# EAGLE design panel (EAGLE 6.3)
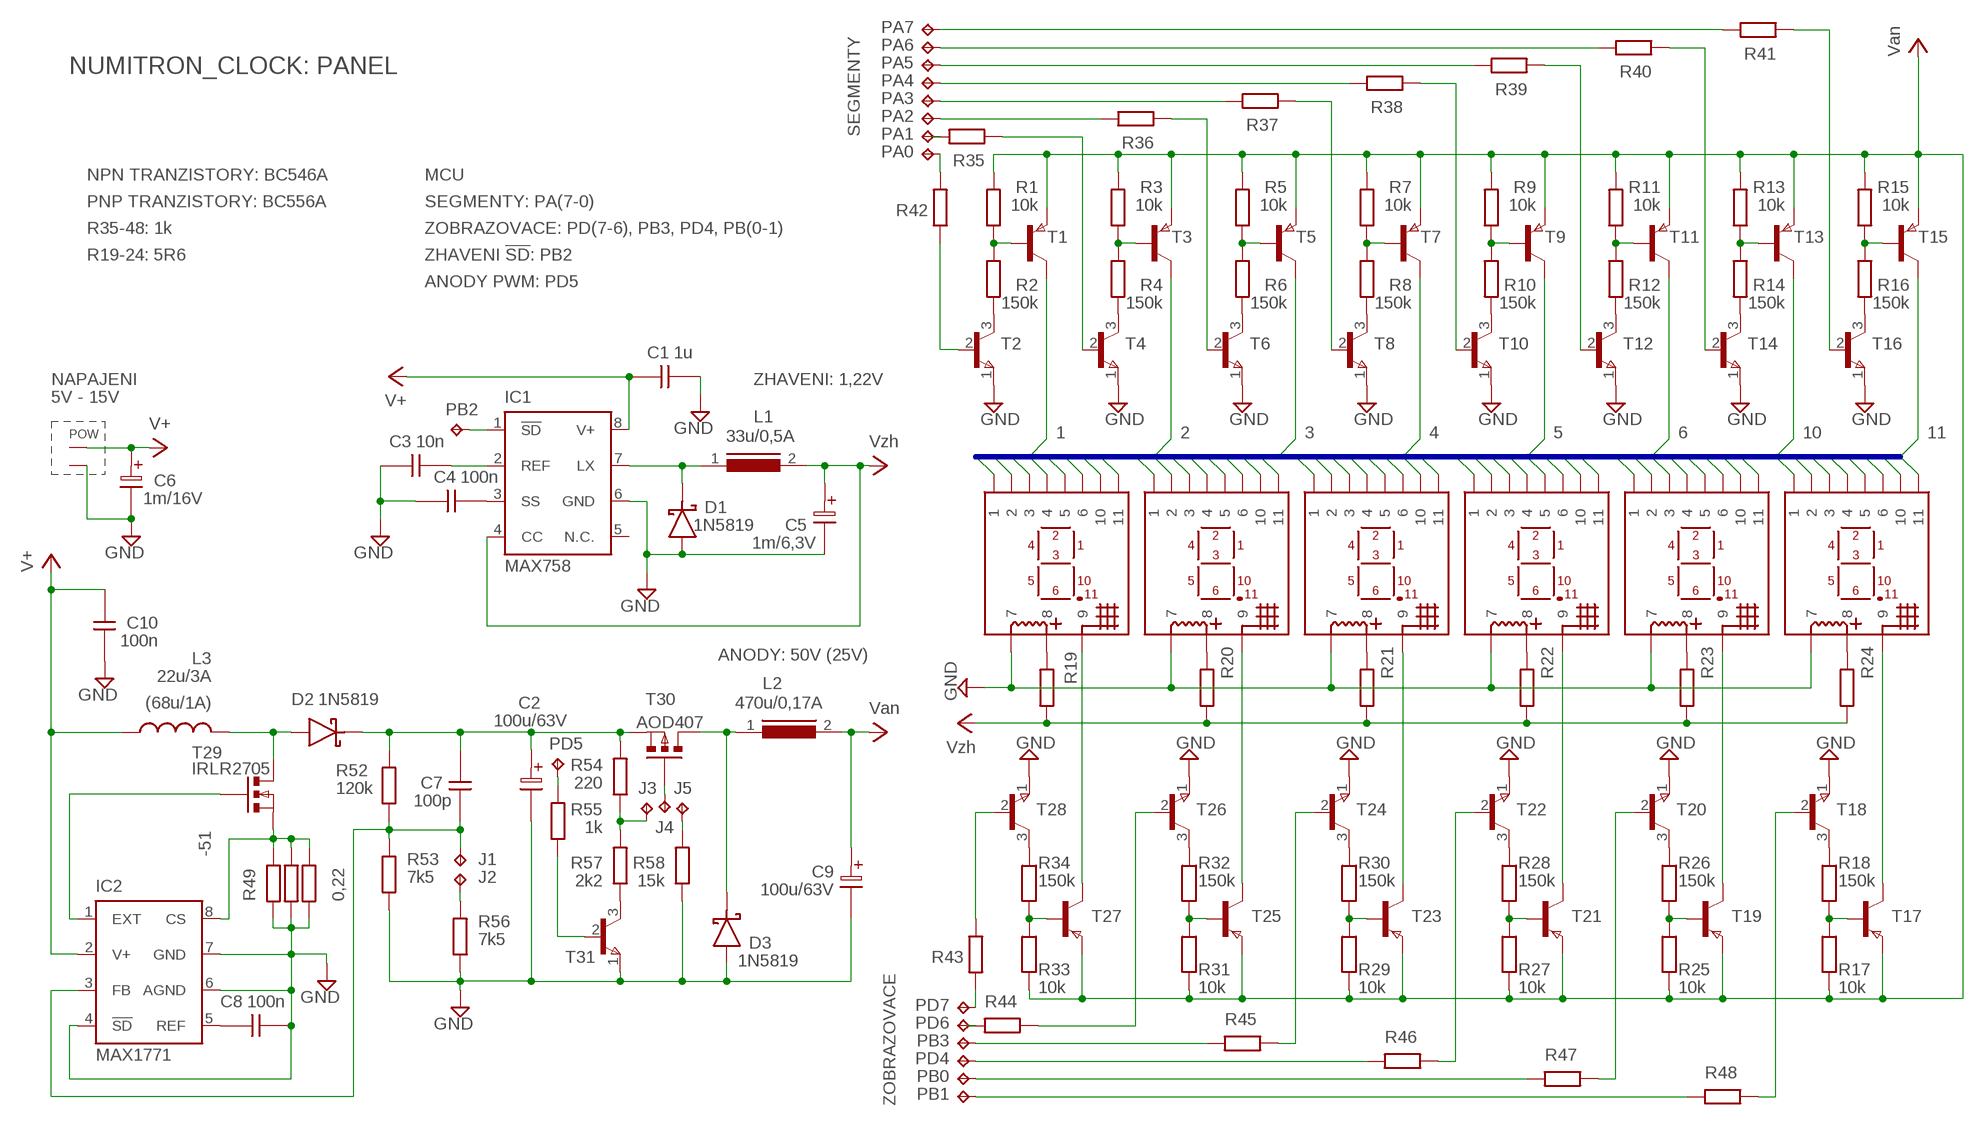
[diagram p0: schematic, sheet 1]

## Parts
C1  1u  CK  [CK]
C2  100u/63V  CT15  [CT15]
C3  10n  CK  [CK]
C4  100n  CK  [CK]
C5  1m/6,3V  CT15  [CT15]
C6  1m/16V  CT15  [CT15]
C7  100p  CK  [CK]
C8  100n  CK  [CK]
C9  100u/63V  CT15  [CT15]
C10  100n  CK  [CK]
D1  1N5819  [DO41]
D2  1N5819  [DO41]
D3  1N5819  [DO41]
DIGIT1  IV6  [IV6]
DIGIT2  IV6  [IV6]
DIGIT3  IV6  [IV6]
DIGIT4  IV6  [IV6]
DIGIT5  IV6  [IV6]
DIGIT6  IV6  [IV6]
IC1  MAX758  [DIL08]
IC2  MAX1771  [DIL08]
J1  TPPAD1-13Y  [P1-13Y]
J2  TPPAD1-13Y  [P1-13Y]
J3  TPPAD1-13Y  [P1-13Y]
J4  TPPAD1-13Y  [P1-13Y]
J5  TPPAD1-13Y  [P1-13Y]
L1  33u/0,5A  SMCC12  [SMCC12]
L2  470u/0,17A  SMCC12  [SMCC12]
L3  22u/3A  TOR.  [L_14X8]
PA0  TPPAD1-13Y  [P1-13Y]
PA1  TPPAD1-13Y  [P1-13Y]
PA2  TPPAD1-13Y  [P1-13Y]
PA3  TPPAD1-13Y  [P1-13Y]
PA4  TPPAD1-13Y  [P1-13Y]
PA5  TPPAD1-13Y  [P1-13Y]
PA6  TPPAD1-13Y  [P1-13Y]
PA7  TPPAD1-13Y  [P1-13Y]
PB0  TPPAD1-13Y  [P1-13Y]
PB1  TPPAD1-13Y  [P1-13Y]
PB2  TPPAD1-13Y  [P1-13Y]
PB3  TPPAD1-13Y  [P1-13Y]
PD4  TPPAD1-13Y  [P1-13Y]
PD5  TPPAD1-13Y  [P1-13Y]
PD6  TPPAD1-13Y  [P1-13Y]
PD7  TPPAD1-13Y  [P1-13Y]
POW  ARK500/2  [ARK500/2]
R1  10k  MRRB  [MRR_1206]
R2  150k  MRRB  [MRR_1206]
R3  10k  MRRB  [MRR_1206]
R4  150k  MRRB  [MRR_1206]
R5  10k  MRRB  [MRR_1206]
R6  150k  MRRB  [MRR_1206]
R7  10k  MRRB  [MRR_1206]
R8  150k  MRRB  [MRR_1206]
R9  10k  MRRB  [MRR_1206]
R10  150k  MRRB  [MRR_1206]
R11  10k  MRRB  [MRR_1206]
R12  150k  MRRB  [MRR_1206]
R13  10k  MRRB  [MRR_1206]
R14  150k  MRRB  [MRR_1206]
R15  10k  MRRB  [MRR_1206]
R16  150k  MRRB  [MRR_1206]
R17  10k  MRRB  [MRR_1206]
R18  150k  MRRB  [MRR_1206]
R19  MRRB  [MRR_1206]
R20  MRR'  [MRR]
R21  MRR'  [MRR]
R22  MRRA  [MRR_0204/10]
R23  MRRA  [MRR_0204/10]
R24  MRRA  [MRR_0204/10]
R25  10k  MRRB  [MRR_1206]
R26  150k  MRRB  [MRR_1206]
R27  10k  MRRB  [MRR_1206]
R28  150k  MRRB  [MRR_1206]
R29  10k  MRRB  [MRR_1206]
R30  150k  MRRB  [MRR_1206]
R31  10k  MRRB  [MRR_1206]
R32  150k  MRRB  [MRR_1206]
R33  10k  MRRB  [MRR_1206]
R34  150k  MRRB  [MRR_1206]
R35  MRR'  [MRR]
R36  MRR'  [MRR]
R37  MRR'  [MRR]
R38  MRR'  [MRR]
R39  MRR'  [MRR]
R40  MRR'  [MRR]
R41  MRR'  [MRR]
R42  MRR'  [MRR]
R43  MRR'  [MRR]
R44  MRR'  [MRR]
R45  MRR'  [MRR]
R46  MRR'  [MRR]
R47  MRR'  [MRR]
R48  MRR'  [MRR]
R49  0,22  MRR-10  [RR-10]
R50  0,22  MRR-10  [RR-10]
R51  0,22  MRR-10  [RR-10]
R52  120k  MRR'  [MRR]
R53  7k5  MRR'  [MRR]
R54  220  MRR'  [MRR]
R55  1k  MRR'  [MRR]
R56  7k5  MRR'  [MRR]
R57  2k2  MRR'  [MRR]
R58  15k  MRR'  [MRR]
T1  BC556  BC556A  [TO-92C]
T2  BC546  BC546A  [TO-92C]
T3  BC546  BC556A  [TO-92C]
T4  BC546  BC546A  [TO-92C]
T5  BC546  BC556A  [TO-92C]
T6  BC546  BC546A  [TO-92C]
T7  BC546  BC556A  [TO-92C]
T8  BC546  BC546A  [TO-92C]
T9  BC546  BC556A  [TO-92C]
T10  BC546  BC546A  [TO-92C]
T11  BC546  BC556A  [TO-92C]
T12  BC546  BC546A  [TO-92C]
T13  BC546  BC556A  [TO-92C]
T14  BC546  BC546A  [TO-92C]
T15  BC546  BC556A  [TO-92C]
T16  BC546  BC546A  [TO-92C]
T17  BC546  BC556A  [TO-92C]
T18  BC546  BC546A  [TO-92C]
T19  BC546  BC556A  [TO-92C]
T20  BC546  BC546A  [TO-92C]
T21  BC546  BC556A  [TO-92C]
T22  BC546  BC546A  [TO-92C]
T23  BC546  BC556A  [TO-92C]
T24  BC546  BC546A  [TO-92C]
T25  BC546  BC556A  [TO-92C]
T26  BC546  BC546A  [TO-92C]
T27  BC546  BC556A  [TO-92C]
T28  BC546  BC546A  [TO-92C]
T29  IRLR2705  IRF540  [D2PAK]
T30  AOD407  IRF9540  [D2PAK]
T31  BC546  BC546A  [TO-92C]

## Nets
GND: C1.2 C2.2 C3.1 C4.1 C5.2 C6.2 C8.2 C9.2 C10.1 D1.A D3.A DIGIT1.P$7 DIGIT2.P$7 DIGIT3.P$7 DIGIT4.P$7 DIGIT5.P$7 DIGIT6.P$7 IC1.6(GND) IC2.4(!SD) IC2.6(AGND) IC2.7(GND) POW.2 R49.1 R50.1 R51.1 R53.2 R56.2 R58.1 T2.1(E) T4.1(E) T6.1(E) T8.1(E) T10.1(E) T12.1(E) T14.1(E) T16.1(E) T18.1(E) T20.1(E) T22.1(E) T24.1(E) T26.1(E) T28.1(E) T31.1(E)
N$1: R1.1 R2.2 T1.2(B)
N$2: R2.1 T2.3(C)
N$3: J2.TP R56.1
N$4: R3.1 R4.2 T3.2(B)
N$5: R4.1 T4.3(C)
N$6: PA0.TP R42.1
N$7: R5.1 R6.2 T5.2(B)
N$8: R6.1 T6.3(C)
N$9: PA1.TP R35.2
N$10: R7.1 R8.2 T7.2(B)
N$11: R8.1 T8.3(C)
N$12: PA2.TP R36.2
N$13: R9.1 R10.2 T9.2(B)
N$14: R10.1 T10.3(C)
N$15: PA3.TP R37.2
N$16: R11.1 R12.2 T11.2(B)
N$17: R12.1 T12.3(C)
N$18: PA4.TP R38.2
N$19: R13.1 R14.2 T13.2(B)
N$20: R14.1 T14.3(C)
N$21: PA5.TP R39.2
N$22: R15.1 R16.2 T15.2(B)
N$23: R16.1 T16.3(C)
N$24: PA6.TP R40.2
N$25: R17.1 R18.2 T17.2(B)
N$26: R18.1 T18.3(C)
N$27: PA7.TP R41.2
N$28: IC2.8(CS) R49.2 R50.2 R51.2 T29.S
N$29: DIGIT1.P$8 R19.2
N$30: DIGIT2.P$8 R20.2
N$31: DIGIT3.P$8 R21.2
N$32: DIGIT4.P$8 R22.2
N$33: DIGIT5.P$8 R23.2
N$34: DIGIT6.P$8 R24.2
N$35: IC1.1(!SD) PB2.TP
N$36: R25.1 R26.2 T19.2(B)
N$37: R26.1 T20.3(C)
N$38: R35.1 T4.2(B)
N$39: R27.1 R28.2 T21.2(B)
N$40: R28.1 T22.3(C)
N$41: R36.1 T6.2(B)
N$42: R29.1 R30.2 T23.2(B)
N$43: R30.1 T24.3(C)
N$44: R37.1 T8.2(B)
N$45: R31.1 R32.2 T25.2(B)
N$46: R32.1 T26.3(C)
N$47: R38.1 T10.2(B)
N$48: R33.1 R34.2 T27.2(B)
N$49: R34.1 T28.3(C)
N$50: R39.1 T12.2(B)
N$51: DIGIT6.P$9 T17.3(C)
N$52: DIGIT5.P$9 T19.3(C)
N$53: DIGIT4.P$9 T21.3(C)
N$54: DIGIT3.P$9 T23.3(C)
N$55: DIGIT2.P$9 T25.3(C)
N$56: DIGIT1.P$9 T27.3(C)
N$57: R40.1 T14.2(B)
N$58: R42.2 T2.2(B)
N$59: R41.1 T16.2(B)
N$60: PD7.TP R43.2
N$61: R43.1 T28.2(B)
N$62: PD6.TP R44.1
N$63: PB3.TP R45.1
N$64: PD4.TP R46.1
N$65: PB0.TP R47.1
N$66: PB1.TP R48.1
N$67: R48.2 T18.2(B)
N$68: R47.2 T20.2(B)
N$69: R46.2 T22.2(B)
N$70: R45.2 T24.2(B)
N$71: R44.2 T26.2(B)
N$72: J5.TP R58.2
N$73: C4.2 IC1.3(SS)
N$74: D1.K IC1.7(LX) L1.1
N$75: C3.2 IC1.2(REF)
N$76: IC2.1(EXT) T29.G
N$77: R55.1 T31.2(B)
N$78: D2.A L3.P$4 T29.D
N$79: C7.1 IC2.3(FB) J1.TP R52.2 R53.1
N$80: C2.1 C7.2 D2.K R52.1 R54.2 T30.S
N$81: D3.K L2.1 T30.D
N$82: J4.TP T30.G
N$83: R57.1 T31.3(C)
N$84: PD5.TP R55.2
N$85: J3.TP R54.1 R57.2
N$87: C8.1 IC2.5(REF)
SEGMENTY0: DIGIT1.P$1 DIGIT2.P$1 DIGIT3.P$1 DIGIT4.P$1 DIGIT5.P$1 DIGIT6.P$1 T1.3(C)
SEGMENTY1: DIGIT1.P$2 DIGIT2.P$2 DIGIT3.P$2 DIGIT4.P$2 DIGIT5.P$2 DIGIT6.P$2 T3.3(C)
SEGMENTY2: DIGIT1.P$3 DIGIT2.P$3 DIGIT3.P$3 DIGIT4.P$3 DIGIT5.P$3 DIGIT6.P$3 T5.3(C)
SEGMENTY3: DIGIT1.P$4 DIGIT2.P$4 DIGIT3.P$4 DIGIT4.P$4 DIGIT5.P$4 DIGIT6.P$4 T7.3(C)
SEGMENTY4: DIGIT1.P$5 DIGIT2.P$5 DIGIT3.P$5 DIGIT4.P$5 DIGIT5.P$5 DIGIT6.P$5 T9.3(C)
SEGMENTY5: DIGIT1.P$6 DIGIT2.P$6 DIGIT3.P$6 DIGIT4.P$6 DIGIT5.P$6 DIGIT6.P$6 T11.3(C)
SEGMENTY6: DIGIT1.P$10 DIGIT2.P$10 DIGIT3.P$10 DIGIT4.P$10 DIGIT5.P$10 DIGIT6.P$10 T13.3(C)
SEGMENTY7: DIGIT1.P$11 DIGIT2.P$11 DIGIT3.P$11 DIGIT4.P$11 DIGIT5.P$11 DIGIT6.P$11 T15.3(C)
V+: C1.1 C6.1 C10.2 IC1.8(V+) IC2.2(V+) L3.P$3 POW.1
VAN: C9.1 L2.2 R1.2 R3.2 R5.2 R7.2 R9.2 R11.2 R13.2 R15.2 R17.2 R25.2 R27.2 R29.2 R31.2 R33.2 T1.1(E) T3.1(E) T5.1(E) T7.1(E) T9.1(E) T11.1(E) T13.1(E) T15.1(E) T17.1(E) T19.1(E) T21.1(E) T23.1(E) T25.1(E) T27.1(E) ; supply symbol labelled Van
VZH: C5.1 IC1.4(CC) L1.2 R19.1 R20.1 R21.1 R22.1 R23.1 R24.1 ; supply symbol labelled Vzh
Unconnected: IC1.5(N.C.)

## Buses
SEGMENTY[0..7]

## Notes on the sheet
- NUMITRON_CLOCK: PANEL
- SEGMENTY
- NPN TRANZISTORY: BC546A | MCU
- PNP TRANZISTORY: BC556A | SEGMENTY: PA(7-0)
- R35-48: 1k | ZOBRAZOVACE: PD(7-6), PB3, PD4, PB(0-1)
- R19-24: 5R6 | ZHAVENI !SD!: PB2
- ANODY PWM: PD5
- NAPAJENI | ZHAVENI: 1,22V
- 5V - 15V
- 1 | 2 | 3 | 4 | 5 | 6 | 10 | 11
- ANODY: 50V (25V)
- (68u/1A)
- -51
- ZOBRAZOVACE

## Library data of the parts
C1 C3 C4 C7 C8 C10 = #_GM99:CK
C2 C5 C6 C9 = #_GM99:CT15: RM = 5mm, R = 10mm
D1-D3 = #_GM99:1N5819
DIGIT1-DIGIT6 = #_my:IV6
IC1 = #_my:MAX758
IC2 = #_my:MAX1771
J1-J5 PA0 PA1-PA7 PB0 PB1-PB3 PD4-PD7 = testpad:TP: Test pad
L1 L2 = inductors:SMCC12: INDUCTOR
L3 = #_my:TOR.
POW = #_GM99:ARK500/2
R1-R48 R52-R58 = #_GM99:MRR
R49-R51 = #_GM99:MRR-10
T1 T3 T5 T7 T9 T11 T13 T15 T17 T19 T21 T23 T25 T27 = #_GM99:BC556A
T2 T4 T6 T8 T10 T12 T14 T16 T18 T20 T22 T24 T26 T28 T31 = #_GM99:BC546A
T29 = #_my:IRF540
T30 = #_my:IRF9540

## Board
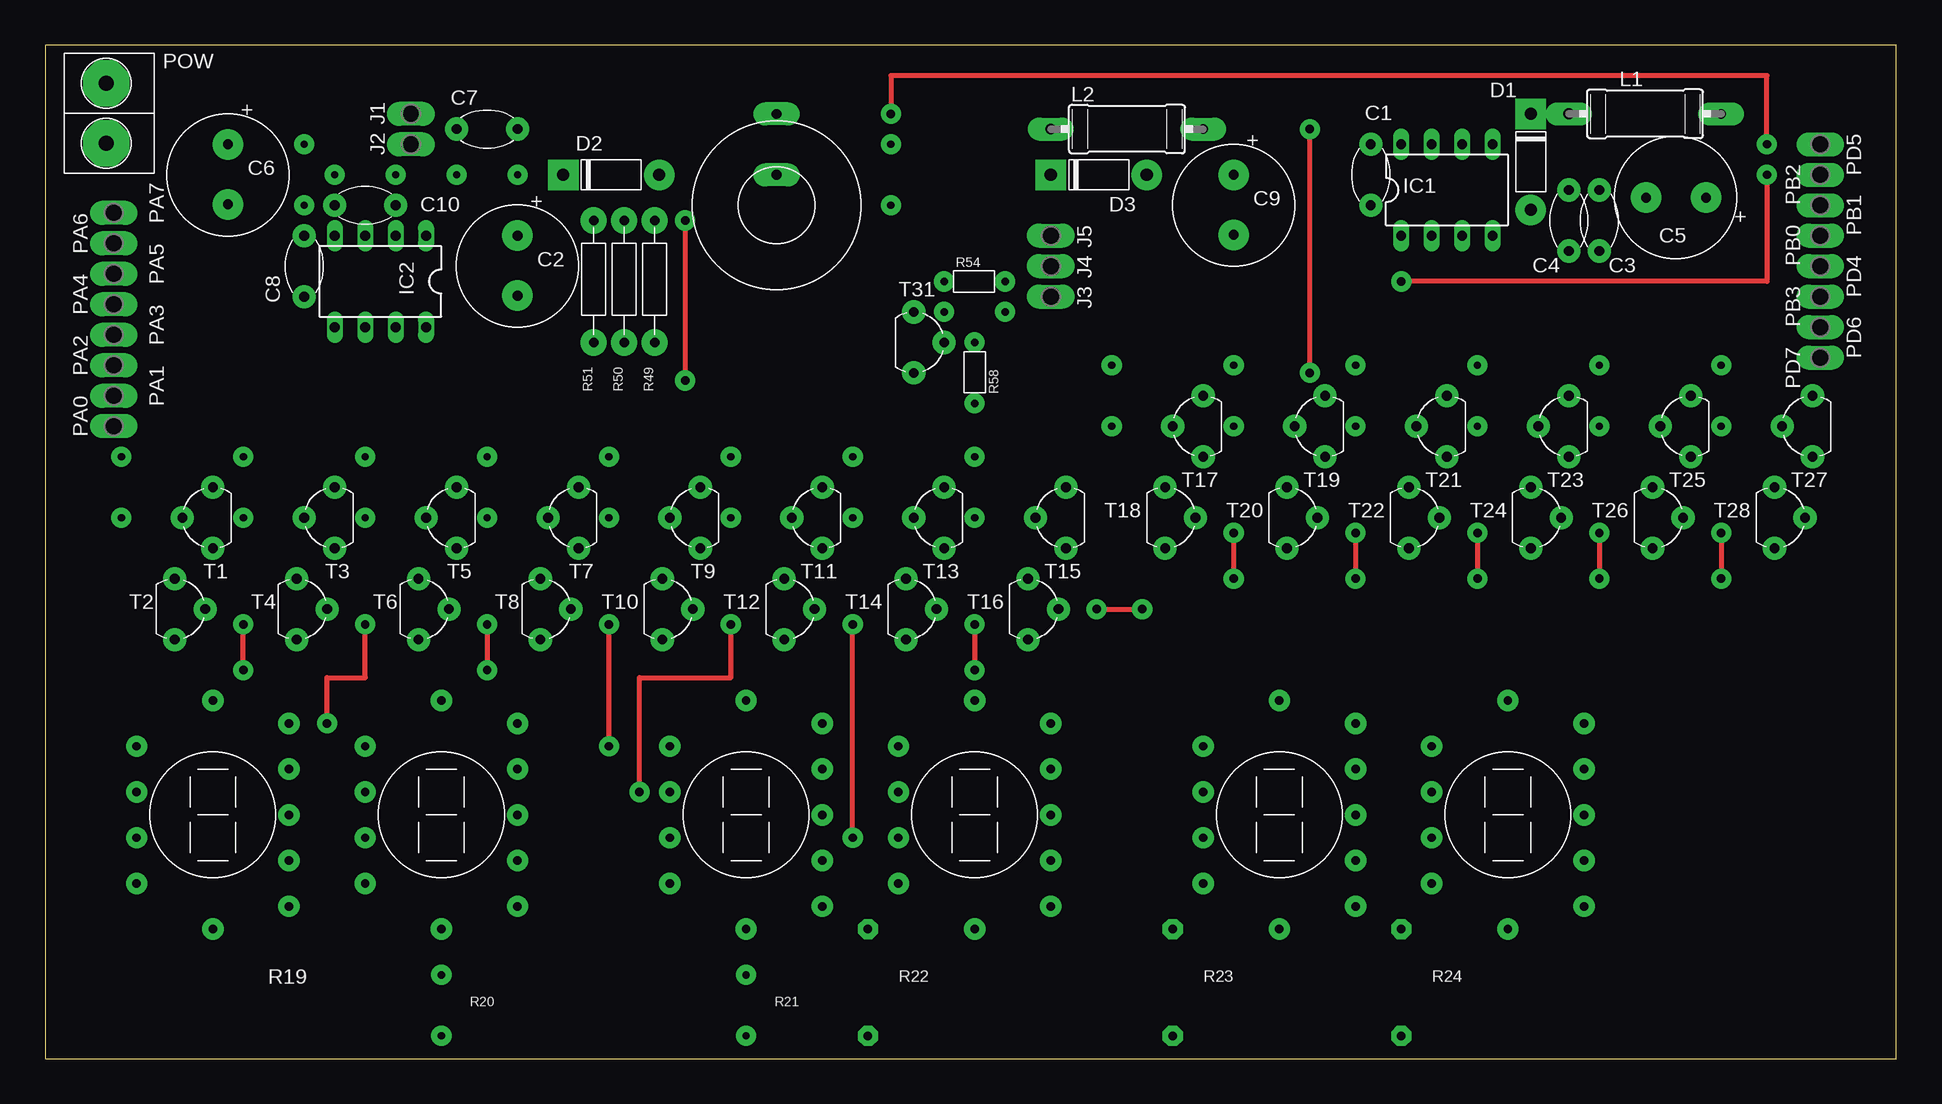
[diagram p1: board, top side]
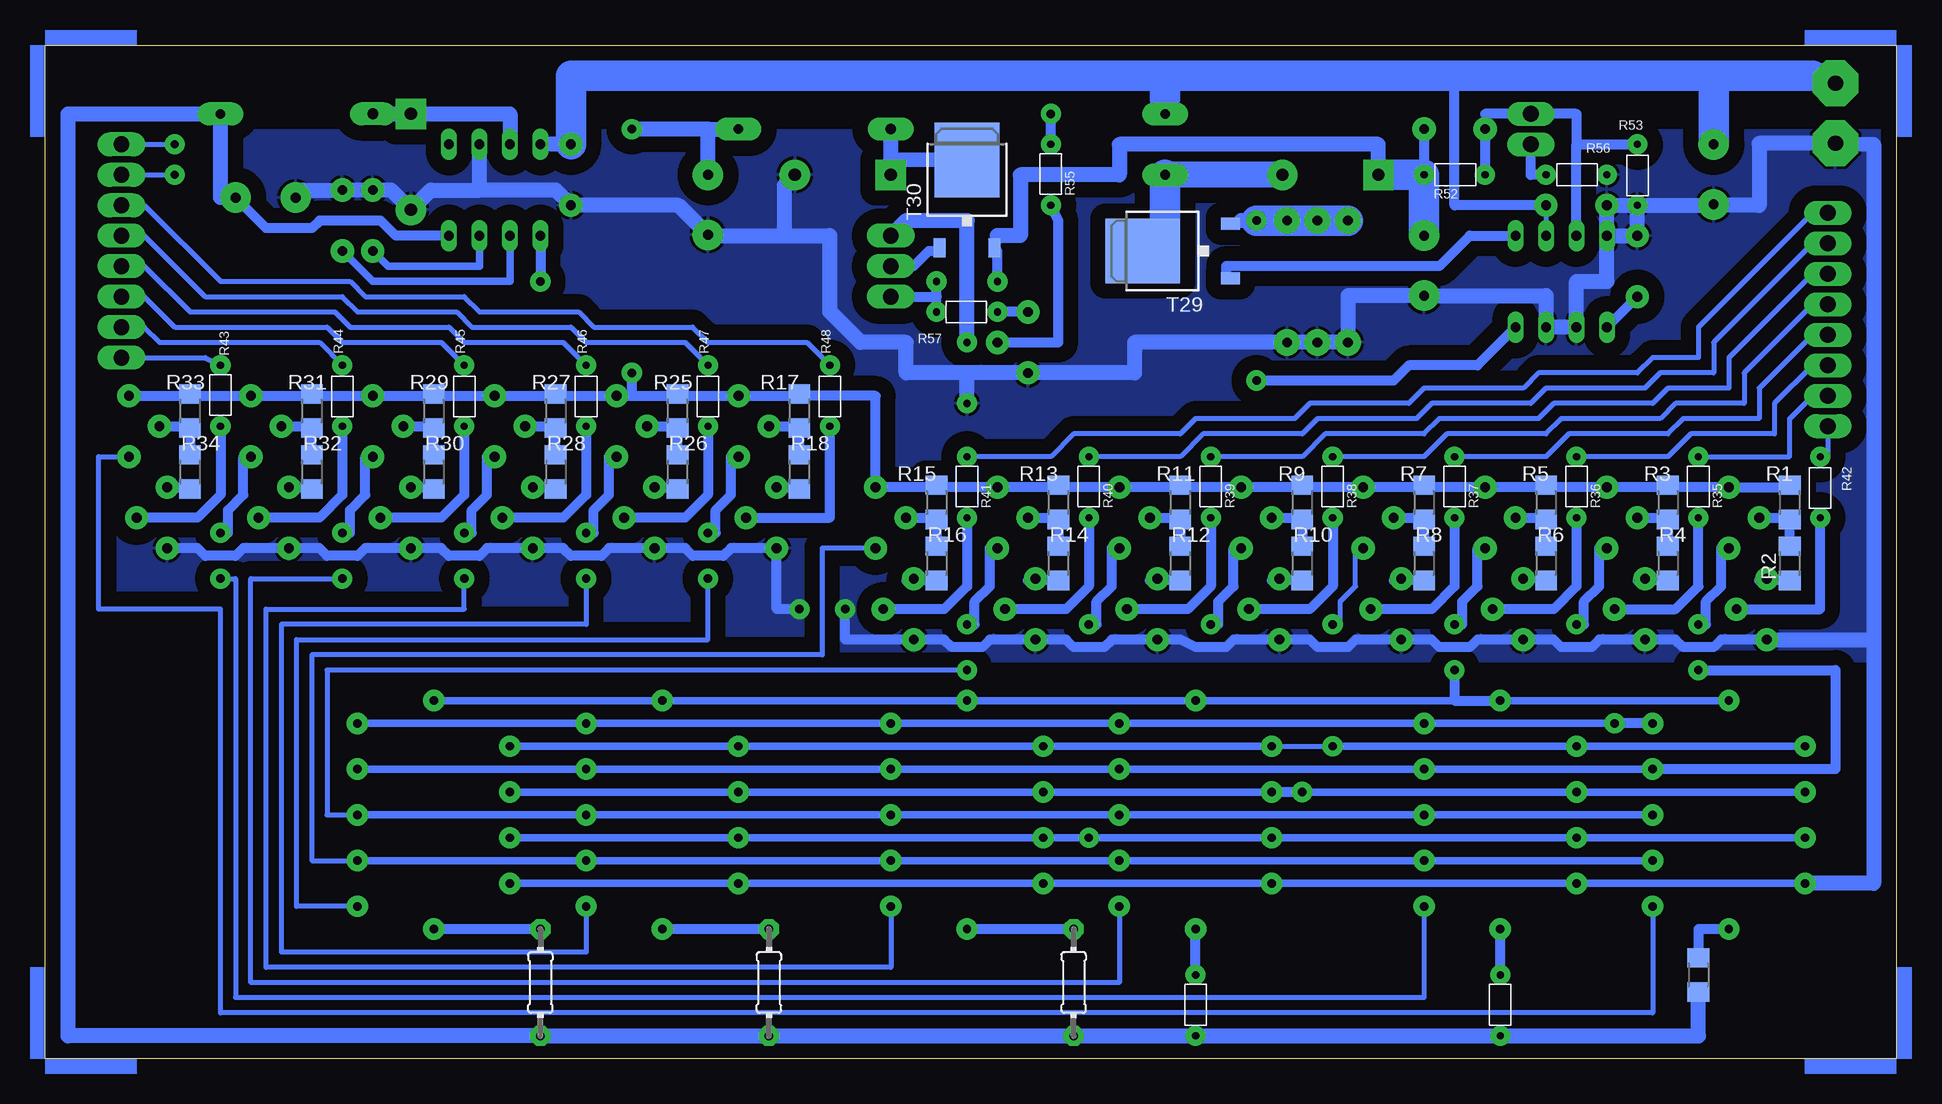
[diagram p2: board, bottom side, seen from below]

Size 154.31 x 84.45 mm. Coordinates in mm from the lower left corner, seen from the top.
Outline: 0,0 154.31,0 154.31,84.45 0,84.45 0,0
Copper layers (1*16): Top 0.035mm / dielectric 1.5mm / Bottom 0.035mm
Design rules "default": minimum track width 10mil, minimum drill 24mil, track to track 8mil, track to pad 8mil, pad to pad 8mil, via to via 8mil, smd to smd 8mil, copper to edge 40mil, drill to drill 8mil, minimum pad ring 10mil, minimum via ring 8mil, stop-mask expansion 4mil, vias tented up to drill 0mil, thermal gap 10mil

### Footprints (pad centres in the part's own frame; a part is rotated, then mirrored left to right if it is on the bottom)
CK = drill 0.813 pad 1.93: 1 0,0; 2 5.08,0
CT15 = drill 0.813 pad 2.54: 1 0,0; 2 5,0
DO41 = drill 1.016 pad 2.54: A 8,0 | drill 1.016 pad 2.54 square: K 0,0
IV6 = drill 0.7 pad 1.778: P$1 6.35,3.81; P$2 6.35,7.62; P$3 0,9.525; P$4 -6.35,5.715; P$5 -6.35,1.905; P$6 -6.35,-1.905; P$7 -6.35,-5.715; P$8 0,-9.525; P$9 6.35,-7.62; P$10 6.35,0; P$11 6.35,-3.81
DIL08 = drill 0.813 long: 1 -3.81,-3.81; 2 -1.27,-3.81; 3 1.27,-3.81; 4 3.81,-3.81; 5 3.81,3.81; 6 1.27,3.81; 7 -1.27,3.81; 8 -3.81,3.81
P1-13Y = drill 1.321 pad 1.905 long: TP 0,0
SMCC12 = drill 0.9 pad 1.93 long: 1 -6.35,0 | drill 0.8 pad 1.93 long: 2 6.35,0
L_14X8 = drill 0.8 pad 1.93 long: P$3 0,7.62; P$4 0,2.54
ARK500/2 = drill 1.27 pad 3.81 octagon: 1 0,0; 2 5,0
MRR_1206 = smd 1.6 x 1.803: 1 -1.422,0; 2 1.422,0
MRR = drill 0.61 pad 1.676: 1 0,0; 2 5.08,0
MRR_0204/10 = drill 0.7 pad 1.676 octagon: 1 -4.445,0; 2 4.445,0
RR-10 = drill 0.8 pad 2.184: 1 0,0; 2 10.16,0
TO-92C = drill 0.813 pad 1.93: 1 0,-1.27; 2 2.54,1.27; 3 0,3.81
D2PAK = smd 5.4 x 6.2: D 0,1.23 | smd 1 x 1.6: G -2.28,-6.07; S 2.28,-6.07

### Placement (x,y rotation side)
C1  110.49,76.2 270 top
C2  39.37,68.58 270 top
C3  129.54,72.39 270 top
C4  127,72.39 270 top
C5  138.43,71.75 180 top
C6  15.24,76.2 270 top
C7  34.29,77.47 0 top
C8  21.59,63.5 90 top
C9  99.06,73.66 270 top
C10  24.13,71.12 0 top
D1  123.83,78.74 270 top
D2  43.18,73.66 0 top
D3  83.82,73.66 0 top
DIGIT1  13.97,20.32 0 top
DIGIT2  33.02,20.32 0 top
DIGIT3  58.42,20.32 0 top
DIGIT4  77.47,20.32 0 top
DIGIT5  102.87,20.32 0 top
DIGIT6  121.92,20.32 0 top
IC1  116.84,72.39 0 top
IC2  27.94,64.77 180 top
J1  30.48,78.74 90 top
J2  30.48,76.2 90 top
J3  83.82,63.5 270 top
J4  83.82,66.04 270 top
J5  83.82,68.58 270 top
L1  133.35,78.74 0 top
L2  90.17,77.47 0 top
L3  60.96,71.12 0 top
PA0  5.71,52.7 90 top
PA1  5.71,55.24 90 top
PA2  5.71,57.78 90 top
PA3  5.71,60.33 90 top
PA4  5.71,62.87 90 top
PA5  5.71,65.41 90 top
PA6  5.71,67.94 90 top
PA7  5.71,70.48 90 top
PB0  147.96,68.58 270 top
PB1  147.96,71.12 270 top
PB2  147.96,73.66 270 top
PB3  147.96,63.5 270 top
PD4  147.96,66.04 270 top
PD5  147.96,76.2 270 top
PD6  147.96,60.96 270 top
PD7  147.96,58.42 270 top
POW  5.08,81.28 270 top
R1  8.89,46.35 90 bottom
R2  8.89,41.27 90 bottom
R3  19.05,46.35 90 bottom
R4  19.05,41.27 90 bottom
R5  29.21,46.35 90 bottom
R6  29.21,41.27 90 bottom
R7  39.37,46.35 90 bottom
R8  39.37,41.27 90 bottom
R9  49.53,46.35 90 bottom
R10  49.53,41.27 90 bottom
R11  59.69,46.35 90 bottom
R12  59.69,41.27 90 bottom
R13  69.85,46.35 90 bottom
R14  69.85,41.27 90 bottom
R15  80.01,46.35 90 bottom
R16  80.01,41.27 90 bottom
R17  91.44,53.98 90 bottom
R18  91.44,48.9 90 bottom
R19  16.51,6.99 90 bottom
R20  33.02,1.91 90 bottom
R21  58.42,1.91 90 bottom
R22  68.58,6.35 90 bottom
R23  93.98,6.35 90 bottom
R24  113.03,6.35 90 bottom
R25  101.6,53.98 90 bottom
R26  101.6,48.9 90 bottom
R27  111.76,53.98 90 bottom
R28  111.76,48.9 90 bottom
R29  121.92,53.98 90 bottom
R30  121.92,48.9 90 bottom
R31  132.08,53.98 90 bottom
R32  132.08,48.9 90 bottom
R33  142.24,53.98 90 bottom
R34  142.24,48.9 90 bottom
R35  16.51,45.09 90 bottom
R36  26.67,45.09 90 bottom
R37  36.83,45.09 90 bottom
R38  46.99,45.09 90 bottom
R39  57.15,45.09 90 bottom
R40  67.31,45.09 90 bottom
R41  77.47,45.09 90 bottom
R42  6.35,50.16 270 bottom
R43  139.7,52.7 90 bottom
R44  129.54,57.78 270 bottom
R45  119.38,57.78 270 bottom
R46  109.22,57.78 270 bottom
R47  99.06,57.78 270 bottom
R48  88.9,57.78 270 bottom
R49  50.8,59.69 90 top
R50  48.26,59.69 90 top
R51  45.72,59.69 90 top
R52  39.37,73.66 0 bottom
R53  21.59,76.2 270 bottom
R54  80.01,64.77 180 top
R55  70.48,71.12 90 bottom
R56  29.21,73.66 0 bottom
R57  74.93,62.23 180 bottom
R58  77.47,54.61 90 top
T1  13.97,46.35 180 top
T2  10.79,36.2 0 top
T3  24.13,46.35 180 top
T4  20.95,36.2 0 top
T5  34.29,46.35 180 top
T6  31.11,36.2 0 top
T7  44.45,46.35 180 top
T8  41.27,36.2 0 top
T9  54.61,46.35 180 top
T10  51.44,36.2 0 top
T11  64.77,46.35 180 top
T12  61.59,36.2 0 top
T13  74.93,46.35 180 top
T14  71.75,36.2 0 top
T15  85.09,46.35 180 top
T16  81.92,36.2 0 top
T17  96.52,53.98 180 top
T18  93.34,43.81 0 top
T19  106.68,53.98 180 top
T20  103.5,43.81 0 top
T21  116.84,53.98 180 top
T22  113.67,43.81 0 top
T23  127,53.98 180 top
T24  123.83,43.81 0 top
T25  137.16,53.98 180 top
T26  133.99,43.81 0 top
T27  147.32,53.98 180 top
T28  144.15,43.81 0 top
T29  61.59,67.31 90 bottom
T30  77.47,73.66 0 bottom
T31  72.39,58.42 0 top
U$1  [ANGLE-ARROW-NW1]  0,0 90 top
U$2  [ANGLE-ARROW-NW1]  0,84.45 0 top
U$3  [ANGLE-ARROW-NW1]  154.31,84.45 270 top
U$4  [ANGLE-ARROW-NW1]  154.31,0 180 top

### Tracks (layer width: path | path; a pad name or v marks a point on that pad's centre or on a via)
GND  (via drill 0.7 pad 1.68)
  Top 0.406: v87.63,37.47 v91.44,37.47
  Bottom 0.61: DIGIT1.P$7 DIGIT2.P$7 DIGIT3.P$7 DIGIT4.P$7 DIGIT5.P$7 DIGIT6.P$7
  Bottom 0.813: T28.1 141.6,42.55 140.97,41.91 138.43,41.91 137.79,42.55 T26.1 131.44,42.55 130.81,41.91 128.27,41.91 127.64,42.55 T24.1 121.28,42.55 120.65,41.91 118.11,41.91 117.47,42.55 T22.1 111.12,42.55 110.49,41.91 107.95,41.91 107.31,42.55 T20.1 100.97,42.55 100.33,41.91 97.79,41.91 97.16,42.55 T18.1 93.34,37.47 v91.44,37.47 | T2.1 14.61,34.92 15.24,34.29 17.78,34.29 18.41,34.92 T4.1 24.77,34.92 25.4,34.29 27.94,34.29 28.57,34.92 T6.1 34.92,34.92 35.56,34.29 38.1,34.29 38.73,34.92 T8.1 45.09,34.92 45.72,34.29 48.26,34.29 48.9,34.92 T10.1 55.24,34.92 55.88,34.29 58.42,34.29 59.69,34.92 T12.1 65.41,34.92 66.04,34.29 68.58,34.29 69.22,34.92 T14.1 75.56,34.92 76.2,34.29 78.74,34.29 79.38,34.92 T16.1 87.63,34.92 v87.63,37.47
  Bottom 1.27: T2.1 1.91,34.92 | 1.91,34.92 1.91,14.61 DIGIT1.P$7 | 1.91,34.92 1.91,76.2 POW.2 11.43,76.28 11.43,71.12 15.24,71.12 | R53.2 15.24,71.12 | 15.24,71.12 C6.2 | R53.2 C10.1 IC2.4 | R53.2 C8.2 IC2.4 | IC2.4 24.13,64.77 26.67,64.77 IC2.6 IC2.7 29.21,63.58 C2.2 45.72,63.58 R51.1 R50.1 R49.1 63.5,59.69 63.5,57.15 T31.1 77.47,57.15 | 77.47,57.15 82.55,57.15 82.55,59.69 86.36,59.69 88.9,62.23 88.9,68.58 92.71,68.58 | D3.A 92.71,72.77 92.71,68.58 | 92.71,68.58 98.98,68.58 C9.2 101.52,71.12 C1.2 111.76,72.39 118.11,72.39 | 118.11,72.39 IC1.6 | 118.11,72.39 122.17,72.39 D1.A 125.47,72.39 C4.1 C3.1 132.79,72.39 C5.2 | R58.1 77.47,57.15
  pour Bottom (isolate 1.27): 1.27,77.47 152.4,77.47 152.4,33.02 1.27,33.02
N$1
  Bottom 0.406: 8.89,45.09 R1.1
  Bottom 0.813: T1.2 8.89,45.09 | R2.2 R1.1
N$2
  Bottom 0.813: R2.1 11.43,39.85 T2.3
N$3
  Bottom 0.813: R56.1 30.48,73.66 J2.TP
N$4
  Bottom 0.813: T3.2 19.05,45.09 R3.1 R4.2
N$5
  Bottom 0.406: 21.59,39.85 T4.3
  Bottom 0.813: R4.1 21.59,39.85
N$6
  Bottom 0.406: PA0.TP 5.71,50.16 R42.1
N$7
  Bottom 0.813: T5.2 29.21,45.09 R5.1 R6.2
N$8
  Bottom 0.406: R6.1 31.75,39.85 T6.3
N$9
  Bottom 0.406: R35.2 8.89,50.16 8.89,53.34 6.99,55.24 PA1.TP
N$10
  Bottom 0.813: T7.2 39.37,45.09 R7.1 R8.2
N$11
  Bottom 0.406: 41.91,39.85 T8.3
  Bottom 0.813: R8.1 41.91,39.85
N$12
  Bottom 0.406: PA2.TP 6.99,57.78 10.16,54.61 10.16,52.07 17.14,52.07 19.05,50.16 R36.2
N$13
  Bottom 0.813: T9.2 49.53,45.09 R9.1 49.53,44.45 R10.2
N$14
  Bottom 0.406: 52.07,39.85 T10.3
  Bottom 0.813: R10.1 52.07,39.85
N$15
  Bottom 0.406: PA3.TP 6.99,60.33 11.43,55.88 11.43,53.34 17.78,53.34 19.05,52.07 27.3,52.07 29.21,50.16 R37.2
N$16
  Bottom 0.813: T11.2 59.69,45.09 R11.1 59.69,44.45 R12.2
N$17
  Bottom 0.406: 62.23,39.85 T12.3
  Bottom 0.813: R12.1 62.23,39.85
N$18
  Bottom 0.406: PA4.TP 6.99,62.87 12.7,57.15 12.7,54.61 18.41,54.61 19.68,53.34 27.94,53.34 29.21,52.07 37.47,52.07 39.37,50.16 R38.2
N$19
  Bottom 0.813: T13.2 69.85,45.09 R13.1 69.85,44.45 R14.2
N$20
  Bottom 0.406: 72.39,39.85 T14.3
  Bottom 0.813: R14.1 72.39,39.85
N$21
  Bottom 0.406: PA5.TP 6.99,65.41 13.97,58.42 13.97,55.88 19.05,55.88 20.32,54.61 28.57,54.61 29.84,53.34 38.1,53.34 39.37,52.07 47.62,52.07 49.53,50.16 R39.2
N$22
  Bottom 0.813: T15.2 80.01,45.09 R15.1 R16.2
N$23
  Bottom 0.406: 82.55,39.85 T16.3
  Bottom 0.813: R16.1 82.55,39.85
N$24
  Bottom 0.406: PA6.TP 6.99,67.94 15.24,59.69 15.24,57.15 19.68,57.15 20.95,55.88 29.21,55.88 30.48,54.61 38.73,54.61 40.01,53.34 48.26,53.34 49.53,52.07 57.78,52.07 59.69,50.16 R40.2
N$25
  Bottom 0.406: 91.44,52.7 R17.1
  Bottom 0.813: R18.2 R17.1 | T17.2 91.44,52.7
N$26
  Bottom 0.813: T18.3 91.44,47.62 R18.1
N$27
  Bottom 0.406: PA7.TP 6.99,70.48 16.51,60.96 16.51,58.42 20.32,58.42 21.59,57.15 29.84,57.15 31.11,55.88 39.37,55.88 40.64,54.61 48.9,54.61 50.16,53.34 58.42,53.34 59.69,52.07 68.58,52.07 70.48,50.16 R41.2
N$28  (via drill 0.7 pad 1.68)
  Top 0.406: v53.34,69.85 v53.34,56.52
  Bottom 0: 54.61,69.85 T29.S
  Bottom 0.813: IC2.8 34.92,57.78 40.64,57.78 41.91,56.52 v53.34,56.52
  Bottom 1.27: v53.34,69.85 54.61,69.85
  Bottom 2.54: R51.2 R50.2 R49.2 v53.34,69.85
N$29
  Bottom 0.813: DIGIT1.P$8 16.51,10.79 R19.2
N$30
  Bottom 0.813: R20.2 DIGIT2.P$8
N$31
  Bottom 0.813: R21.2 DIGIT3.P$8
N$32
  Bottom 0.813: R22.2 DIGIT4.P$8
N$33
  Bottom 0.813: R23.2 DIGIT5.P$8
N$34
  Bottom 0.813: R24.2 DIGIT6.P$8
N$35  (via drill 0.7 pad 1.68)
  Top 0.406: v113.03,64.77 143.51,64.77 v143.51,73.66
  Bottom 0.406: PB2.TP v143.51,73.66
  Bottom 0.813: IC1.1 v113.03,64.77
N$36
  Bottom 0.406: 101.6,52.7 R25.1
  Bottom 0.813: R26.2 R25.1 | T19.2 101.6,52.7
N$37
  Bottom 0.406: 101.6,47.62 R26.1
  Bottom 0.813: T20.3 101.6,47.62
N$38
  Bottom 0.813: T4.2 18.41,37.47 16.51,39.37 R35.1
N$39
  Bottom 0.406: 111.76,52.7 R27.1
  Bottom 0.813: R28.2 R27.1 | T21.2 111.76,52.7
N$40
  Bottom 0.406: 111.76,47.62 R28.1
  Bottom 0.813: T22.3 111.76,47.62
N$41
  Bottom 0.813: R36.1 26.67,39.37 28.57,37.47 T6.2
N$42
  Bottom 0.406: 121.92,52.7 R29.1
  Bottom 0.813: R30.2 R29.1 | T23.2 121.92,52.7
N$43
  Bottom 0.406: 121.92,47.62 R30.1
  Bottom 0.813: T24.3 121.92,47.62
N$44
  Bottom 0.813: R37.1 36.83,39.37 38.73,37.47 T8.2
N$45
  Bottom 0.406: 132.08,52.7 R31.1
  Bottom 0.813: R32.2 R31.1 | T25.2 132.08,52.7
N$46
  Bottom 0.406: 132.08,47.62 R32.1
  Bottom 0.813: T26.3 132.08,47.62
N$47
  Bottom 0.813: R38.1 46.99,39.37 48.9,37.47 T10.2
N$48
  Bottom 0.406: 142.24,52.7 R33.1
  Bottom 0.813: T27.2 142.24,52.7 | R33.1 R34.2
N$49
  Bottom 0.406: 142.24,47.62 R34.1
  Bottom 0.813: T28.3 142.24,47.62
N$50
  Bottom 0.813: R39.1 57.15,39.37 59.05,37.47 T12.2
N$51  (via drill 0.7 pad 1.68)
  Top 0.406: v99.06,43.81 v99.06,40.01
  Bottom 0.406: DIGIT6.P$9 133.35,12.7 133.35,34.92 99.06,34.92 v99.06,40.01
  Bottom 0.813: v99.06,43.81 98.42,43.81 98.42,45.72 97.16,46.99 97.16,50.16 T17.3
N$52  (via drill 0.7 pad 1.68)
  Top 0.406: v109.22,43.81 v109.22,40.01
  Bottom 0.406: DIGIT5.P$9 109.22,8.89 134.62,8.89 134.62,36.2 109.22,36.2 v109.22,40.01
  Bottom 0.813: v109.22,43.81 108.58,43.81 108.58,45.72 107.31,46.99 107.31,50.16 T19.3
N$53  (via drill 0.7 pad 1.68)
  Top 0.406: v119.38,43.81 v119.38,40.01
  Bottom 0.406: DIGIT4.P$9 83.82,7.62 135.89,7.62 135.89,37.47 119.38,37.47 v119.38,40.01
  Bottom 0.813: v119.38,43.81 118.75,43.81 118.75,45.72 117.47,46.99 117.47,50.16 T21.3
N$54  (via drill 0.7 pad 1.68)
  Top 0.406: v129.54,43.81 v129.54,40.01
  Bottom 0.406: DIGIT3.P$9 64.77,6.35 137.16,6.35 137.16,40.01 v129.54,40.01
  Bottom 0.813: v129.54,43.81 128.91,43.81 128.91,45.72 127.64,46.99 127.64,50.16 T23.3
N$55  (via drill 0.7 pad 1.68)
  Top 0.406: v139.7,43.81 v139.7,40.01
  Bottom 0.406: DIGIT2.P$9 39.37,5.08 138.43,5.08 138.43,40.01 v139.7,40.01
  Bottom 0.813: v139.7,43.81 139.06,43.81 139.06,45.72 137.79,46.99 137.79,50.16 T25.3
N$56
  Bottom 0.406: DIGIT1.P$9 20.32,3.81 139.7,3.81 139.7,37.47 149.86,37.47 149.86,50.16 T27.3
N$57
  Bottom 0.813: R40.1 67.31,39.37 69.22,37.47 T14.2
N$58
  Bottom 0.813: T2.2 6.35,37.47 R42.2
N$59
  Bottom 0.813: R41.1 77.47,39.37 79.38,37.47 T16.2
N$60
  Bottom 0.406: PD7.TP 140.97,58.42 R43.2
N$61
  Bottom 0.813: R43.1 139.7,46.99 141.6,45.09 T28.2
N$62
  Bottom 0.406: PD6.TP 146.05,60.96 144.78,59.69 131.44,59.69 R44.1
N$63
  Bottom 0.406: PB3.TP 146.05,63.5 143.51,60.96 130.81,60.96 129.54,59.69 121.28,59.69 R45.1
N$64
  Bottom 0.406: PD4.TP 146.05,66.04 142.24,62.23 130.18,62.23 128.91,60.96 120.65,60.96 119.38,59.69 111.12,59.69 R46.1
N$65
  Bottom 0.406: PB0.TP 146.05,68.58 140.97,63.5 129.54,63.5 128.27,62.23 120.02,62.23 118.75,60.96 110.49,60.96 109.22,59.69 100.97,59.69 R47.1
N$66
  Bottom 0.406: PB1.TP 146.05,71.12 139.7,64.77 128.91,64.77 127.64,63.5 119.38,63.5 118.11,62.23 109.86,62.23 108.58,60.96 100.33,60.96 99.06,59.69 90.81,59.69 R48.1
N$67
  Bottom 0.813: T18.2 88.9,45.09 R48.2
N$68
  Bottom 0.813: R47.2 99.06,46.99 100.97,45.09 T20.2
N$69
  Bottom 0.813: R46.2 109.22,46.99 111.12,45.09 T22.2
N$70
  Bottom 0.813: R45.2 119.38,46.99 121.28,45.09 T24.2
N$71
  Bottom 0.813: R44.2 129.54,46.99 131.44,45.09 T26.2
N$72
  Bottom 1.27: R58.2 77.47,69.85 82.55,69.85 J5.TP
N$73
  Bottom 0.61: C4.2 125.73,66.04 118.11,66.04 IC1.3
N$74
  Bottom 1.27: L1.1 D1.K 115.57,78.74 IC1.7
N$75
  Bottom 0.61: IC1.2 115.57,64.77 127,64.77 C3.2
N$76
  Bottom 0.813: T29.G 55.88,65.41 55.88,66.04 38.1,66.04 35.56,68.58 IC2.1
N$77
  Bottom 0.813: T31.2 69.85,59.69 69.85,69.85 R55.1
N$78
  Bottom 0.406: 60.96,67.31 T29.D
  Bottom 2.184: D2.A L3.P$4
  Bottom 2.54: L3.P$4 60.96,67.31
N$79
  Bottom 0.406: 34.29,78.74 C7.1
  Bottom 0.813: C7.1 R52.2 | 34.29,78.74 J1.TP 26.67,78.74 26.67,76.2 | IC2.3 26.67,76.2 | 26.67,76.2 R53.1
N$80
  Bottom 0.406: 74.93,67.31 T30.S
  Bottom 0.813: C7.2 R52.1 | 74.93,68.58 T30.S | R54.2 74.93,67.31
  Bottom 1.27: D2.K 43.18,76.2 64.77,76.2 64.77,73.66 73.03,73.66 73.03,68.58 74.93,68.58
  Bottom 2.54: C2.1 R52.1 D2.K
N$81
  Bottom 1.27: D3.K 83.82,74.93 | 83.82,74.93 L2.1 | T30.D 83.82,74.93
N$82
  Bottom 0.813: J4.TP 81.92,66.04 80.64,67.31 80.01,67.31 T30.G
N$83
  Bottom 0.813: T31.3 R57.1
N$84  (via drill 0.7 pad 1.68)
  Top 0.406: v143.51,76.2 143.51,81.92 70.48,81.92 v70.48,78.74
  Bottom 0.406: PD5.TP v143.51,76.2
  Bottom 0.813: R55.2 v70.48,78.74
N$85
  Bottom 0.813: R57.2 80.01,63.5 | 80.01,63.5 R54.1 | J3.TP 80.01,63.5
N$87
  Bottom 0.813: C8.1 IC2.5
SEGMENTY0  (via drill 0.7 pad 1.68)
  Top 0.406: v16.51,32.38 v16.51,36.2
  Bottom 0.406: 14.61,42.55 T1.3
  Bottom 0.61: DIGIT1.P$1 DIGIT2.P$1 DIGIT3.P$1 DIGIT4.P$1 DIGIT5.P$1 DIGIT6.P$1
  Bottom 0.813: v16.51,32.38 5.08,32.38 5.08,24.13 DIGIT1.P$1 | v16.51,36.2 15.88,36.2 15.88,38.1 14.61,39.37 14.61,42.55
SEGMENTY1  (via drill 0.7 pad 1.68)
  Top 0.406: v23.5,27.94 23.5,31.75 26.67,31.75 v26.67,36.2
  Bottom 0.61: DIGIT6.P$2 DIGIT5.P$2 DIGIT4.P$2 DIGIT3.P$2 DIGIT2.P$2 v23.5,27.94
  Bottom 0.813: v26.67,36.2 26.04,36.2 26.04,38.1 24.77,39.37 24.77,42.55 T3.3 | DIGIT1.P$2 v23.5,27.94
SEGMENTY2  (via drill 0.7 pad 1.68)
  Top 0.406: v36.83,36.2 v36.83,32.38
  Bottom 0.61: DIGIT6.P$3 DIGIT5.P$3 DIGIT4.P$3 DIGIT3.P$3 36.83,29.84 | DIGIT2.P$3 DIGIT1.P$3
  Bottom 0.813: DIGIT2.P$3 36.83,29.84 v36.83,32.38 | v36.83,36.2 36.2,36.2 36.2,38.1 34.92,39.37 34.92,42.55 T5.3
SEGMENTY3  (via drill 0.7 pad 1.68)
  Top 0.406: v46.99,26.04 v46.99,36.2
  Bottom 0.406: v46.99,36.2 46.35,36.2 46.35,38.1 45.09,39.37 45.09,42.55 T7.3 | DIGIT3.P$4 v46.99,26.04
  Bottom 0.61: DIGIT1.P$4 DIGIT2.P$4 v46.99,26.04 | DIGIT3.P$4 DIGIT4.P$4 DIGIT5.P$4 DIGIT6.P$4
SEGMENTY4  (via drill 0.7 pad 1.68)
  Top 0.406: v49.53,22.23 49.53,31.75 57.15,31.75 v57.15,36.2
  Bottom 0.61: DIGIT6.P$5 DIGIT5.P$5 DIGIT4.P$5 DIGIT3.P$5 | v49.53,22.23 DIGIT2.P$5 DIGIT1.P$5
  Bottom 0.813: v57.15,36.2 56.52,36.2 56.52,38.1 55.24,39.37 55.24,42.55 T9.3 | v49.53,22.23 DIGIT3.P$5
SEGMENTY5  (via drill 0.7 pad 1.68)
  Top 0.406: v67.31,18.41 v67.31,36.2
  Bottom 0.61: DIGIT1.P$6 DIGIT2.P$6 DIGIT3.P$6 v67.31,18.41 DIGIT4.P$6 DIGIT5.P$6 DIGIT6.P$6
  Bottom 0.813: v67.31,36.2 66.67,36.2 66.67,38.1 65.41,39.37 65.41,42.55 T11.3
SEGMENTY6  (via drill 0.7 pad 1.68)
  Top 0.406: v77.47,36.2 v77.47,32.38
  Bottom 0.406: v77.47,32.38 130.81,32.38 130.81,20.32 DIGIT6.P$10
  Bottom 0.61: DIGIT6.P$10 DIGIT5.P$10 DIGIT4.P$10 DIGIT3.P$10 DIGIT2.P$10 DIGIT1.P$10
  Bottom 0.813: v77.47,36.2 76.83,36.2 76.83,38.1 75.56,39.37 75.56,42.55 T13.3
SEGMENTY7
  Bottom 0.406: T15.3 89.53,42.55 89.53,33.66 132.08,33.66 132.08,16.51 DIGIT6.P$11
  Bottom 0.61: DIGIT1.P$11 DIGIT2.P$11 DIGIT3.P$11 DIGIT4.P$11 DIGIT5.P$11 DIGIT6.P$11
V+
  Bottom 0.406: C10.2 IC2.2
  Bottom 0.813: C10.2 36.83,71.12 36.83,81.92
  Bottom 1.27: C1.1 IC1.8 | 60.96,80.01 L3.P$3
  Bottom 2.54: POW.1 6.99,81.92 15.24,81.92 | 15.24,81.92 36.83,81.92 60.96,81.92 | C6.1 15.24,81.92 | 60.96,81.92 110.49,81.92 C1.1 | 60.96,81.92 60.96,80.01
VAN  (via drill 0.7 pad 1.68)
  Top 0.406: v105.41,57.15 v105.41,77.47
  Bottom 0.406: 8.89,47.62 R1.2 | R5.2 29.21,47.62 | R7.2 39.37,47.62 | R9.2 49.53,47.62 | R11.2 59.69,47.62 | R13.2 69.85,47.62 | R15.2 80.01,47.62 | R3.2 19.05,47.62 | 92.08,55.24 R17.2 90.81,55.24 | R25.2 101.6,55.24 | R27.2 111.76,55.24 | R29.2 121.92,55.24 | R31.2 132.08,55.24 | R33.2 142.24,55.24
  Bottom 0.813: 8.89,47.62 T1.1 19.05,47.62 T3.1 29.21,47.62 T5.1 39.37,47.62 T7.1 49.53,47.62 T9.1 59.69,47.62 T11.1 69.85,47.62 T13.1 80.01,47.62 T15.1 85.09,55.24 90.81,55.24 | T27.1 142.24,55.24 T25.1 132.08,55.24 T23.1 121.92,55.24 T21.1 111.76,55.24 T19.1 105.41,55.24 | 105.41,55.24 101.6,55.24 T17.1 92.08,55.24 | v105.41,57.15 105.41,55.24
  Bottom 1.27: C9.1 99.06,77.47 | 99.06,77.47 L2.2 | 99.06,77.47 v105.41,77.47
VZH
  Bottom 0.813: IC1.4 125.09,68.58 126.36,69.85 131.44,69.85 132.08,69.22 135.89,69.22 C5.1
  Bottom 1.27: R19.1 16.51,1.91 R20.1 R21.1 R22.1 R23.1 R24.1 152.4,1.91 152.4,78.74 L1.2 139.7,71.75 C5.1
